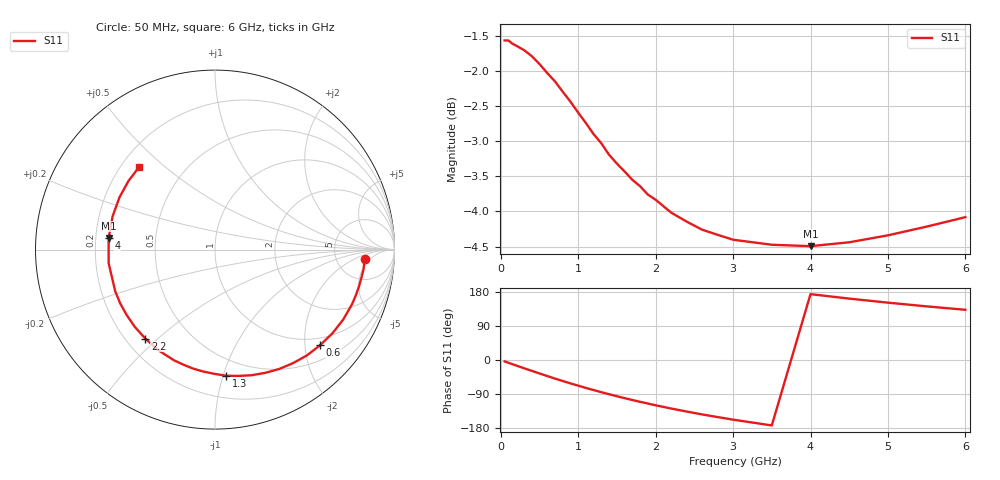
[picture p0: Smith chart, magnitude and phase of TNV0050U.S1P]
! SIEMENS Discrete & RF Semiconductors
! BAS70-07W
! Si Schottky Diode in SOT343
! IF = 0.05 mA
! S-Parameters:  February  1997
# GHz  S  MA  R  50
!  f  S11
! GHz  MAG  ANG
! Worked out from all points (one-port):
!   34 points, 50 MHz to 6 GHz, reference 50 ohm
!   lowest |S11| = -4.5 dB at 4 GHz (marker M1), VSWR 3.95, Z = 12.7 + j2.53 ohm
!   |S11| at or under -10 dB: nowhere
!   S11 on the Smith chart (normalised r, x): 50 MHz: 10, -4; 600 MHz: 0.82, -2.34; 1.3 GHz: 0.37, -1.02; 2.2 GHz: 0.28, -0.46; 4 GHz: 0.25, +0.05; 6 GHz: 0.27, +0.41
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0.05  0.835 -3.7
0.15  0.8306 -11.0
0.3  0.8219 -21.7
0.4  0.8139 -28.6
0.5  0.8034 -35.5
0.6  0.7916 -42.3
0.7  0.7809 -49.0
0.8  0.7678 -55.4
0.9  0.7553 -61.7
1  0.7418 -67.7
1.1  0.7292 -73.7
1.3  0.7053 -85.0
1.5  0.6824 -95.6
1.6  0.6736 -100.7
1.8  0.6575 -110.4
1.9  0.6486 -114.9
2  0.6431 -119.5
2.2  0.6297 -128.0
2.4  0.6205 -136.0
2.6  0.6123 -143.6
2.8  0.6072 -150.6
3  0.6023 -157.4
3.5  0.5974 -172.7
4  0.596 173.8
4.5  0.5998 162.0
5  0.6067 151.3
5.5  0.6154 141.5
6  0.625 132.5
